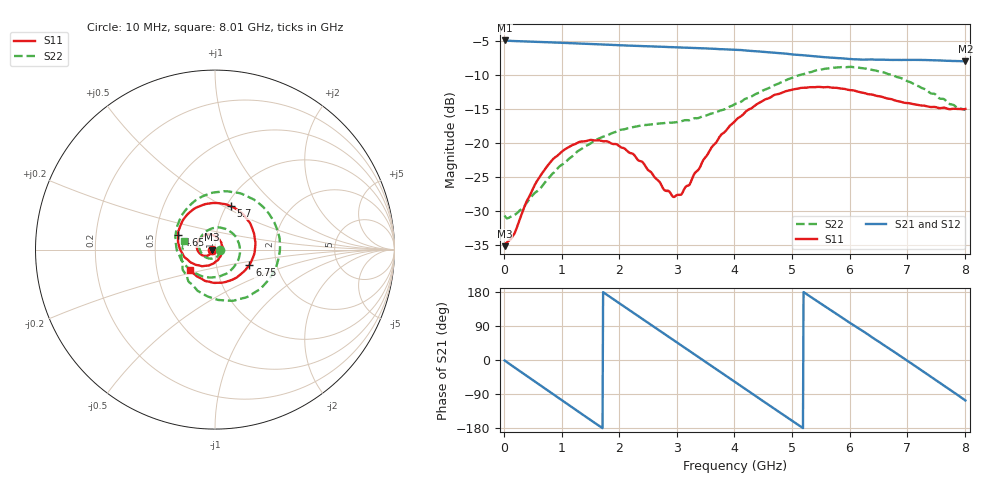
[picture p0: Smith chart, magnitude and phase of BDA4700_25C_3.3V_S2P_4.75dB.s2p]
!Agilent Technologies,E5071B,MY42404982,A.09.10
!Date: Mon Oct 20 18:04:58 2025
!Data & Calibration Information:
!Freq	S11:SOLT2(ON)	S21:SOLT2(ON)	S12:SOLT2(ON)	S22:SOLT2(ON)
# Hz S RI R 50
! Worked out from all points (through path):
!   801 points, 10 MHz to 8.01 GHz, reference 50 ohm
!   highest |S21| = -4.87 dB at 10 MHz (marker M1); lowest = -7.9 dB at 8.01 GHz (marker M2)
!   group delay of S21, straight-line fit = 286 ps
!   lowest |S11| = -35.1 dB at 10 MHz (marker M3), VSWR 1.04, Z = 48.3 - j0.115 ohm
!   |S11| at or under -10 dB: start of sweep to end of sweep
!   |S22| runs from -31.0 to -8.7 dB; largest |S21 - S12| = 0.0068
!   S11 on the Smith chart (normalised r, x): 10 MHz: 0.97, -0.00; 4.65 GHz: 0.65, +0.11; 5.7 GHz: 1.05, +0.54; 6.75 GHz: 1.45, -0.26; 8.01 GHz: 0.74, -0.17
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1e7  -0.0175 -0.00119  0.5707 -0.0124  0.5707 -0.0127  0.0295 -0.00242
3.3e8  -0.0239 -0.0215  0.4586 -0.3255  0.4581 -0.3258  0.0217 -0.0258
7.1e8  -0.054 -0.0352  0.1397 -0.5367  0.1394 -0.5369  -0.0141 -0.0497
1.02e9  -0.0855 -0.0211  -0.169 -0.5212  -0.1688 -0.5215  -0.0597 -0.0371
1.35e9  -0.1019 0.0162  -0.4291 -0.3297  -0.4293 -0.3299  -0.0889 0.0209
1.93e9  -0.0582 0.08  -0.487 0.205  -0.4869 0.205  -0.00235 0.1211
2.32e9  -0.00365 0.0757  -0.2354 0.464  -0.2355 0.4639  0.0997 0.0892
2.68e9  0.0342 0.0407  0.0919 0.506  0.091 0.5057  0.1392 -0.0117
2.97e9  0.0405 -0.00475  0.3279 0.389  0.3275 0.388  0.1065 -0.095
3.36e9  0.0111 -0.062  0.4945 0.0835  0.495 0.0837  0.00155 -0.1532
4.01e9  -0.1238 -0.0772  0.2594 -0.413  0.2602 -0.4119  -0.1835 -0.0635
4.33e9  -0.1852 -0.0155  -0.00806 -0.4765  -0.00864 -0.4776  -0.22 0.0504
4.65e9  -0.2054 0.0831  -0.2622 -0.384  -0.2612 -0.3852  -0.1907 0.1799
5.01e9  -0.1555 0.1941  -0.4268 -0.1451  -0.4282 -0.1459  -0.069 0.2969
5.35e9  -0.0457 0.2548  -0.4213 0.1212  -0.4218 0.1191  0.106 0.3192
5.7e9  0.0877 0.2412  -0.2671 0.3321  -0.2663 0.3325  0.2766 0.2294
6.17e9  0.2087 0.115  0.0573 0.4095  0.0614 0.4103  0.3588 -0.0229
6.68e9  0.2029 -0.0649  0.3531 0.2103  0.3542 0.2095  0.2058 -0.2488
6.75e9  0.1918 -0.0852  0.3754 0.1657  0.3769 0.163  0.1737 -0.2662
7.28e9  0.0518 -0.1823  0.3533 -0.2087  0.3528 -0.2094  -0.0808 -0.2397
7.65e9  -0.058 -0.1732  0.145 -0.3786  0.1441 -0.379  -0.1808 -0.1067
8.01e9  -0.1395 -0.1126  -0.1159 -0.3838  -0.1149 -0.3844  -0.17 0.0472
